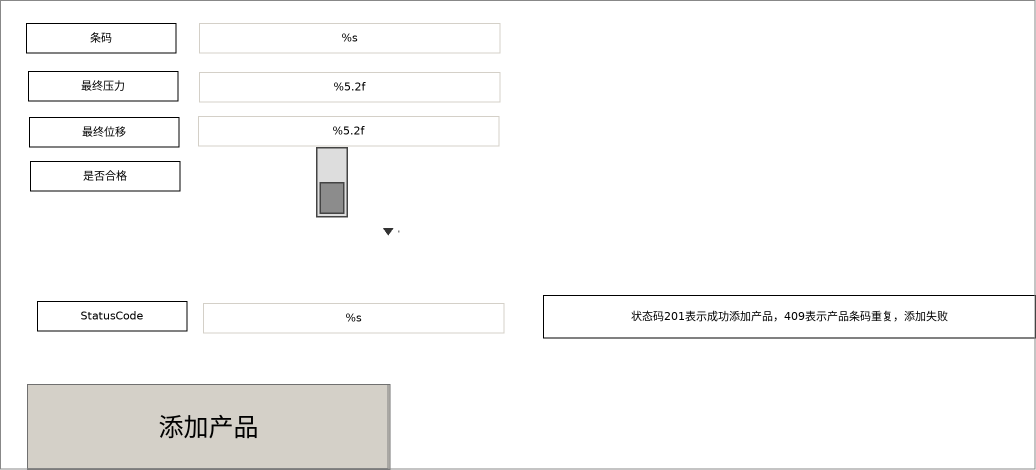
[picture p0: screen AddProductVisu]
VISUALIZATION AddProductVisu  // 1036x470
    ComboBoxInteger (398,231 1x0)
    Rectangle (26,23 150x30), "条码"
    Rectangle (28,71 150x30), "最终压力"
    Rectangle (29,117 150x30), "最终位移"
    Rectangle (30,161 150x30), "是否合格"
    Textfield (199,23 301x30), "%s", text variable: MAIN.fbAddProduct.newProductBarCode
        OnMouseDown: write the text variable via Default
    Textfield (199,72 301x30), "%5.2f", text variable: MAIN.fbAddProduct.newProduct.FinalPressure
        OnMouseDown: write the text variable via Default
    Textfield (198,116 301x30), "%5.2f", text variable: MAIN.fbAddProduct.newProduct.FinalDisplacement
        OnMouseDown: write the text variable via Default
    DipSwitch (297,147 70x70), variable: MAIN.fbAddProduct.newProduct.IsQualified, behaviour: TOGGLE, style: Switch-DipSwitch-Gray
    Button (27,384 363x86), "添加产品"
        tap MAIN.fbAddProduct.bSend
    Rectangle (37,301 150x30), "StatusCode"
    Textfield (203,303 301x30), "%s", text variable: MAIN.fbAddProduct.nStatusCode
        OnMouseDown: write the text variable via Default
    Rectangle (543,295 493x43), "状态码201表示成功添加产品，409表示产品条码重复，添加失败"
END_VISUALIZATION
